ORGANIZATION_BLOCK "MAIN_PROGRAM"
TITLE =
VERSION : 0.1


VAR_TEMP
  OB1_EV_CLASS : BYTE ;	//Bits 0-3 = 1 (Coming event), Bits 4-7 = 1 (Event class 1)
  OB1_SCAN_1 : BYTE ;	//1 (Cold restart scan 1 of OB 1), 3 (Scan 2-n of OB 1)
  OB1_PRIORITY : BYTE ;	//1 (Priority of 1 is lowest)
  OB1_OB_NUMBR : BYTE ;	//1 (Organization block 1, OB1)
  OB1_RESERVED_1 : BYTE ;	//Reserved for system
  OB1_RESERVED_2 : BYTE ;	//Reserved for system
  OB1_PREV_CYCLE : INT ;	//Cycle time of previous OB1 scan (milliseconds)
  OB1_MIN_CYCLE : INT ;	//Minimum cycle time of OB1 (milliseconds)
  OB1_MAX_CYCLE : INT ;	//Maximum cycle time of OB1 (milliseconds)
  OB1_DATE_TIME : DATE_AND_TIME ;	//Date and time OB1 started
END_VAR
BEGIN
NETWORK
TITLE =

      UC    "COPY_OP37_PLC";

      UC    "DB_DB_COPY";

      UC    "TRASFERIMENTO_ACP";

      UC    "INIZIALIZZAZIONE ACP";

      UC    "ANALOG_I/O";

      UC    "COM_GEN";

      UC    "ALARM_MAN";

      UC    "COIL";

      UC    "ASPO";

      UC    "STRAIGHTENER";

      UC    "SVOLG_COILS";

      UC    "ASPO_PRESS_RULLI";

      UC    "COM_MANDRINI_COILS";

      UC    "COM_ SPIANATRICE";

      UC    "COMAND_PEELER";

      UC    "COM_PINCH_ROLLERS";

      UC    "COM_CONPENETRAZ.";

      UC    "COM_GUIDE_BUCA";

      UC    "COM_FEEDER";

      UC    "COM_PASS_LINE";

      UC    "RULLO_ANTI_CADUTA";

      UC    "RULLO_MISURA";

      UC    "COM_CILINDRI_TRASCIN.";

      UC    "FOTO_PRES_LAMIERA";

      UC    "RULLI_GUIDA_INF";

END_ORGANIZATION_BLOCK

